|Texas Instruments Incorporated
| IBIS Model of : TMUX7219
| 48V 2:1 Analog Multiplexer
| This file contains package information for the following:
|  VSSOP 8-pin (DGK) package as [Component] TMUX7219_DGK
|  WSON  8-pin (RQX) package as [Component] TMUX7219_RQX
| This device can be powered at the following Vccs:
| Single Rail Supply Configurations:
|  5.0 volt VDD, 0V VSS
|  12.0 volt VDD, 0V VSS
|  36.0 volt VDD, 0V VSS
|  44.0 volt VDD, 0V VSS
| Dual Rail Supply Configurations:
|  5.0 volt VDD, -5V VSS
|  15.0 volt VDD, -15V VSS
|  20.0 volt VDD, -20V VSS
| Digital Voltage Range : 4.5-48.4
| Package-type: VSSOP 8-pin
| #pins/pkg drawing : 8-pin DGK
[IBIS Ver] 4.1
[File name] tmux7219.ibs
[File Rev] 1.2
[Date] 05/03/2022
[Source]
| Texas Instruments Incorporated.
| 12500 TI Blvd
| Dallas, TX -75243
[Notes] Revision History:
| Rev 1.0: 09/03/2020
| - Initial version of the model
| - Model generated from simulations in TISPICE/SPECTRE
| - C_comp although listed in numerical order of value are
| obtained from varying PVT conditions. For PVT conditions for
| each specific value refer the buffer description under
| respective [Model]. IBIS model user is responsible for using
| appropriate C_comp to simulate for Signal Integrity.
| - Warnings regarding combined Non-monotonicity of various models have been
| reviewed and considered minor and can be ignored.
| Rev 1.1: 01/06/2021
| - Updated Off Leakage Current
| Rev 1.2: 05/03/2022
| - Added RQX package
|**** Modify the following if you use [Model Selector]***********
| - Model names with a trailing voltage extension contain the model for
| operation at that voltage range.
[Disclaimer]
| This model is designed as an aid for customers of Texas Instruments.
| TI and its licensors and suppliers make no warranties, either expressed
| or implied, with respect to this model, including the warranties of
| merchantability or fitness for a particular purpose. The model is
| provided solely on an "as is" basis. The entire risk as to its quality
| and performance is with the customer.
| This model is subject to change without notice. Texas Instruments
| Incorporated is not responsible for updating this model.
[Copyright]
(C) Copyright 2022 Texas Instruments Incorporated. All rights reserved.
| Component TMUX7219_DGK 8-pin SOT (per package)
[Component] TMUX7219_DGK
[Manufacturer]  Texas Instruments Incorporated
[Package] |VSSOP (DGK) 8-pin
| variable typ min max
R_pkg 0.05 0.04 0.06
L_pkg 1.0nH 0.8nH 1.2nH
C_pkg 0.2pF 0.16pF 0.24pF
| pin number (pin name) mapping to model name
[Pin] signal_name   model_name   R_pin L_pin C_pin
1   D   TMUX7219_DX   NA   NA   NA
2   SA   TMUX7219_SX   NA   NA   NA
3   GND   GND   NA   NA   NA
4   VDD   POWER   NA   NA   NA
5   EN   INPUT_PU   NA   NA   NA
6   IN   INPUT_PD   NA   NA   NA
7   VSS   POWER   NA   NA   NA
8   SB   TMUX7219_SX   NA   NA   NA
[Series Switch Groups]
| Function Group States
On  1 /   | SB->D IN HIGH  EN HIGH
   | D->SB IN HIGH  EN HIGH
On  2 /   | SA->D IN LOW   EN HIGH
   | D->SA IN LOW   EN HIGH
Off 1 2 /   | EN LOW
[Series Pin Mapping]   pin_2   model_name   function_table_group
|8   1   TMUX7219_SX_SINGLE_5V_S   1
|1   8   TMUX7219_DX_SINGLE_5V_S   1
|2   1   TMUX7219_SX_SINGLE_5V_S   2
|1   2   TMUX7219_DX_SINGLE_5V_S   2
| 8   1   TMUX7219_SX_SINGLE_12V_S   1
| 1   8   TMUX7219_DX_SINGLE_12V_S   1
| 2   1   TMUX7219_SX_SINGLE_12V_S   2
| 1   2   TMUX7219_DX_SINGLE_12V_S   2
| 8   1   TMUX7219_SX_SINGLE_36V_S   1
| 1   8   TMUX7219_DX_SINGLE_36V_S   1
| 2   1   TMUX7219_SX_SINGLE_36V_S   2
| 1   2   TMUX7219_DX_SINGLE_36V_S   2
| 8   1   TMUX7219_SX_SINGLE_36V_S   1
| 1   8   TMUX7219_DX_SINGLE_36V_S   1
| 2   1   TMUX7219_SX_SINGLE_36V_S   2
| 1   2   TMUX7219_DX_SINGLE_36V_S   2
 8   1   TMUX7219_SX_SINGLE_44V_S   1
 1   8   TMUX7219_DX_SINGLE_44V_S   1
 2   1   TMUX7219_SX_SINGLE_44V_S   2
 1   2   TMUX7219_DX_SINGLE_44V_S   2
| 8   1   TMUX7219_SX_DUAL_PM5_S   1
| 1   8   TMUX7219_DX_DUAL_PM5_S   1
| 2   1   TMUX7219_SX_DUAL_PM5_S   2
| 1   2   TMUX7219_DX_DUAL_PM5_S   2
| 8   1   TMUX7219_SX_DUAL_PM15_S   1
| 1   8   TMUX7219_DX_DUAL_PM15_S   1
| 2   1   TMUX7219_SX_DUAL_PM15_S   2
| 1   2   TMUX7219_DX_DUAL_PM15_S   2
| 8   1   TMUX7219_SX_DUAL_PM20_S   1
| 1   8   TMUX7219_DX_DUAL_PM20_S   1
| 2   1   TMUX7219_SX_DUAL_PM20_S   2
| 1   2   TMUX7219_DX_DUAL_PM20_S   2
| Component TMUX7219_RQX 8-pin SOT (per package)
[Component] TMUX7219_RQX
[Manufacturer]  Texas Instruments Incorporated
[Package] |WSON (RQX) 8-pin
| variable typ min max
R_pkg 0.05 0.04 0.06
L_pkg 1.0nH 0.8nH 1.2nH
C_pkg 0.2pF 0.16pF 0.24pF
| pin number (pin name) mapping to model name
[Pin] signal_name   model_name   R_pin L_pin C_pin
1   D   TMUX7219_DX   NA   NA   NA
2   SA   TMUX7219_SX   NA   NA   NA
3   GND   GND   NA   NA   NA
4   VDD   POWER   NA   NA   NA
5   EN   INPUT_PU   NA   NA   NA
6   IN   INPUT_PD   NA   NA   NA
7   VSS   POWER   NA   NA   NA
8   SB   TMUX7219_SX   NA   NA   NA
[Series Switch Groups]
| Function Group States
|On  1 /   | SB->D IN HIGH  EN HIGH
|   | D->SB IN HIGH  EN HIGH
|On  2 /   | SA->D IN LOW   EN HIGH
|   | D->SA IN LOW   EN HIGH
|Off 1 2 /   | EN LOW
[Series Pin Mapping]   pin_2   model_name   function_table_group
| 8   1   TMUX7219_SX_SINGLE_5V_S   1
| 1   8   TMUX7219_DX_SINGLE_5V_S   1
| 2   1   TMUX7219_SX_SINGLE_5V_S   2
| 1   2   TMUX7219_DX_SINGLE_5V_S   2
| 8   1   TMUX7219_SX_SINGLE_12V_S   1
| 1   8   TMUX7219_DX_SINGLE_12V_S   1
| 2   1   TMUX7219_SX_SINGLE_12V_S   2
| 1   2   TMUX7219_DX_SINGLE_12V_S   2
| 8   1   TMUX7219_SX_SINGLE_36V_S   1
| 1   8   TMUX7219_DX_SINGLE_36V_S   1
| 2   1   TMUX7219_SX_SINGLE_36V_S   2
| 1   2   TMUX7219_DX_SINGLE_36V_S   2
| 8   1   TMUX7219_SX_SINGLE_44V_S   1
| 1   8   TMUX7219_DX_SINGLE_44V_S   1
| 2   1   TMUX7219_SX_SINGLE_44V_S   2
| 1   2   TMUX7219_DX_SINGLE_44V_S   2
| 8   1   TMUX7219_SX_DUAL_PM5_S   1
| 1   8   TMUX7219_DX_DUAL_PM5_S   1
| 2   1   TMUX7219_SX_DUAL_PM5_S   2
| 1   2   TMUX7219_DX_DUAL_PM5_S   2
| 8   1   TMUX7219_SX_DUAL_PM15_S   1
| 1   8   TMUX7219_DX_DUAL_PM15_S   1
| 2   1   TMUX7219_SX_DUAL_PM15_S   2
| 1   2   TMUX7219_DX_DUAL_PM15_S   2
 8   1   TMUX7219_SX_DUAL_PM20_S   1
 1   8   TMUX7219_DX_DUAL_PM20_S   1
 2   1   TMUX7219_SX_DUAL_PM20_S   2
 1   2   TMUX7219_DX_DUAL_PM20_S   2
| Model Selectors
|*** power supply options or driver programmability *********
[Model Selector] INPUT_PU
INBUF_PU_5V   INPUT_PU   buffer at 5V operation.
INBUF_PU_12V   INPUT_PU   buffer at 12V operation.
INBUF_PU_15V   INPUT_PU   buffer at 15V operation.
INBUF_PU_20V   INPUT_PU   buffer at 20V operation.
INBUF_PU_36V   INPUT_PU   buffer at 36V operation.
INBUF_PU_44V   INPUT_PU   buffer at 44V operation.
[Model Selector] INPUT_PD
INBUF_PD_5V   INPUT_PD   buffer at 5V operation.
INBUF_PD_12V   INPUT_PD   buffer at 12V operation.
INBUF_PD_15V   INPUT_PD   buffer at 15V operation.
INBUF_PD_20V   INPUT_PD   buffer at 20V operation.
INBUF_PD_36V   INPUT_PD   buffer at 36V operation.
INBUF_PD_44V   INPUT_PD   buffer at 44V operation.
[Model Selector] TMUX7219_SX
TMUX7219_SX_SINGLE_5V  switch termination at +5V operation.
TMUX7219_SX_SINGLE_12V  switch termination at +12V operation.
TMUX7219_SX_SINGLE_36V  switch termination at +36V operation.
TMUX7219_SX_SINGLE_44V  switch termination at +44V operation.
TMUX7219_SX_DUAL_PM5  switch termination at +/-5V operation.
TMUX7219_SX_DUAL_PM15  switch termination at +/-15V operation.
TMUX7219_SX_DUAL_PM20  switch termination at +/-20V operation.
[Model Selector] TMUX7219_SX_S
TMUX7219_SX_SINGLE_5V_S  switch at +5V operation.
TMUX7219_SX_SINGLE_12V_S  switch at +12V operation.
TMUX7219_SX_SINGLE_36V_S  switch at +36V operation.
TMUX7219_SX_SINGLE_44V_S  switch at +44V operation.
TMUX7219_SX_DUAL_PM5_S  switch at +/-5V operation.
TMUX7219_SX_DUAL_PM15_S  switch at +/-15V operation.
TMUX7219_SX_DUAL_PM20_S  switch at +/-20V operation.
[Model Selector] TMUX7219_DX
TMUX7219_DX_SINGLE_5V  termination switch at +5V operation.
TMUX7219_DX_SINGLE_12V  termination switch at +12V operation.
TMUX7219_DX_SINGLE_36V  termination switch at +36V operation.
TMUX7219_DX_SINGLE_44V  termination switch at +44V operation.
TMUX7219_DX_DUAL_PM5  termination switch at +/-5V operation.
TMUX7219_DX_DUAL_PM15  termination switch at +/-15V operation.
TMUX7219_DX_DUAL_PM20  termination switch at +/-20V operation.
[Model Selector] TMUX7219_DX_S
TMUX7219_DX_SINGLE_5V_S  switch at +5V operation.
TMUX7219_DX_SINGLE_12V_S  switch at +12V operation.
TMUX7219_DX_SINGLE_36V_S  switch at +36V operation.
TMUX7219_DX_SINGLE_44V_S  switch at +44V operation.
TMUX7219_DX_DUAL_PM5_S  switch at +/-5V operation.
TMUX7219_DX_DUAL_PM15_S  switch at +/-15V operation.
TMUX7219_DX_DUAL_PM20_S  switch at +/-20V operation.
[Model]   TMUX7219_SX_SINGLE_5V_S
Model_type  Series_switch
| variable   typ   min   max
C_comp   110pF   110pF   110pF
[Temperature Range]   25   125   -40
| Ambient temperature   25   125   -40
[Voltage range]   5   5   5
[On]
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[Off]
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[Model]   TMUX7219_DX_SINGLE_5V_S
Model_type  Series_switch
| variable   typ   min   max
C_comp   110pF   110pF   110pF
[Temperature Range]   25   125   -40
| Ambient temperature   25   125   -40
[Voltage range]   5   5   5
[On]
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[Off]
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[Model]   TMUX7219_SX_SINGLE_12V_S
Model_type  Series_switch
| variable   typ   min   max
C_comp   155pF   155pF   155pF
[Temperature Range]   25   125   -40
| Ambient temperature   25   125   -40
[Voltage range]   12   12   12
[On]
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[Off]
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[Model]   TMUX7219_DX_SINGLE_12V_S
Model_type  Series_switch
| variable   typ   min   max
C_comp   155pF   155pF   155pF
[Temperature Range]   25   125   -40
| Ambient temperature   25   125   -40
[Voltage range]   12   12   12
[On]
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[Off]
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[Model]   TMUX7219_SX_SINGLE_36V_S
Model_type  Series_switch
| variable   typ   min   max
C_comp   148pF   148pF   148pF
[Temperature Range]   25   125   -40
| Ambient temperature   25   125   -40
[Voltage range]   36   36   36
[On]
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[Off]
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[Model]   TMUX7219_DX_SINGLE_36V_S
Model_type  Series_switch
| variable   typ   min   max
C_comp   148pF   148pF   148pF
[Temperature Range]   25   125   -40
| Ambient temperature   25   125   -40
[Voltage range]   36   36   36
[On]
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[Off]
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[Model]   TMUX7219_SX_SINGLE_44V_S
Model_type  Series_switch
| variable   typ   min   max
C_comp   148pF   148pF   148pF
[Temperature Range]   25   125   -40
| Ambient temperature   25   125   -40
[Voltage range]   44   44   44
[On]
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[Off]
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[Model]   TMUX7219_DX_SINGLE_44V_S
Model_type  Series_switch
| variable   typ   min   max
C_comp   148pF   148pF   148pF
[Temperature Range]   25   125   -40
| Ambient temperature   25   125   -40
[Voltage range]   44   44   44
[On]
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[Off]
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[Model]   TMUX7219_SX_DUAL_PM5_S
Model_type  Series_switch
| variable   typ   min   max
C_comp   120pF   120pF   120pF
[Temperature Range]   25   125   -40
| Ambient temperature   25   125   -40
[Voltage range]   0   -5   5
[On]
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[Off]
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[Model]   TMUX7219_DX_DUAL_PM5_S
Model_type  Series_switch
| variable   typ   min   max
C_comp   120pF   120pF   120pF
[Temperature Range]   25   125   -40
| Ambient temperature   25   125   -40
[Voltage range]   0   -5   5
[On]
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[Off]
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[Model]   TMUX7219_SX_DUAL_PM15_S
Model_type  Series_switch
| variable   typ   min   max
C_comp   150pF   150pF   150pF
[Temperature Range]   25   125   -40
| Ambient temperature   25   125   -40
[Voltage range]   0   -15   15
[On]
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[Off]
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[Model]   TMUX7219_DX_DUAL_PM15_S
Model_type  Series_switch
| variable   typ   min   max
C_comp   150pF   150pF   150pF
[Temperature Range]   25   125   -40
| Ambient temperature   25   125   -40
[Voltage range]   0   -15   15
[On]
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[Off]
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[Model]   TMUX7219_SX_DUAL_PM20_S
Model_type  Series_switch
| variable   typ   min   max
C_comp   148pF   148pF   148pF
[Temperature Range]   25   125   -40
| Ambient temperature   25   125   -40
[Voltage range]   0   -20   20
[On]
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[Off]
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[Model]   TMUX7219_DX_DUAL_PM20_S
Model_type  Series_switch
| variable   typ   min   max
C_comp   148pF   148pF   148pF
[Temperature Range]   25   125   -40
| Ambient temperature   25   125   -40
[Voltage range]   0   -20   20
[On]
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[Off]
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| Models and submodels in the file (40): INBUF_PD_5V (Input), INBUF_PD_12V (Input), INBUF_PD_15V (Input), INBUF_PD_20V (Input), INBUF_PD_36V (Input), INBUF_PD_44V (Input), INBUF_PU_5V (Input), INBUF_PU_12V (Input), INBUF_PU_15V (Input), INBUF_PU_20V (Input), INBUF_PU_36V (Input), INBUF_PU_44V (Input), TMUX7219_SX_SINGLE_5V_S (Series_switch), TMUX7219_SX_SINGLE_5V (Terminator), TMUX7219_DX_SINGLE_5V_S (Series_switch), TMUX7219_DX_SINGLE_5V (Terminator), TMUX7219_SX_SINGLE_12V_S (Series_switch), TMUX7219_SX_SINGLE_12V (Terminator), TMUX7219_DX_SINGLE_12V_S (Series_switch), TMUX7219_DX_SINGLE_12V (Terminator), TMUX7219_SX_SINGLE_36V_S (Series_switch), TMUX7219_SX_SINGLE_36V (Terminator), TMUX7219_DX_SINGLE_36V_S (Series_switch), TMUX7219_DX_SINGLE_36V (Terminator), TMUX7219_SX_SINGLE_44V_S (Series_switch), TMUX7219_SX_SINGLE_44V (Terminator), TMUX7219_DX_SINGLE_44V_S (Series_switch), TMUX7219_DX_SINGLE_44V (Terminator), TMUX7219_SX_DUAL_PM5_S (Series_switch), TMUX7219_SX_DUAL_PM5 (Terminator), TMUX7219_DX_DUAL_PM5_S (Series_switch), TMUX7219_DX_DUAL_PM5 (Terminator), TMUX7219_SX_DUAL_PM15_S (Series_switch), TMUX7219_SX_DUAL_PM15 (Terminator), TMUX7219_DX_DUAL_PM15_S (Series_switch), TMUX7219_DX_DUAL_PM15 (Terminator), TMUX7219_SX_DUAL_PM20_S (Series_switch), TMUX7219_SX_DUAL_PM20 (Terminator), TMUX7219_DX_DUAL_PM20_S (Series_switch), TMUX7219_DX_DUAL_PM20 (Terminator)
